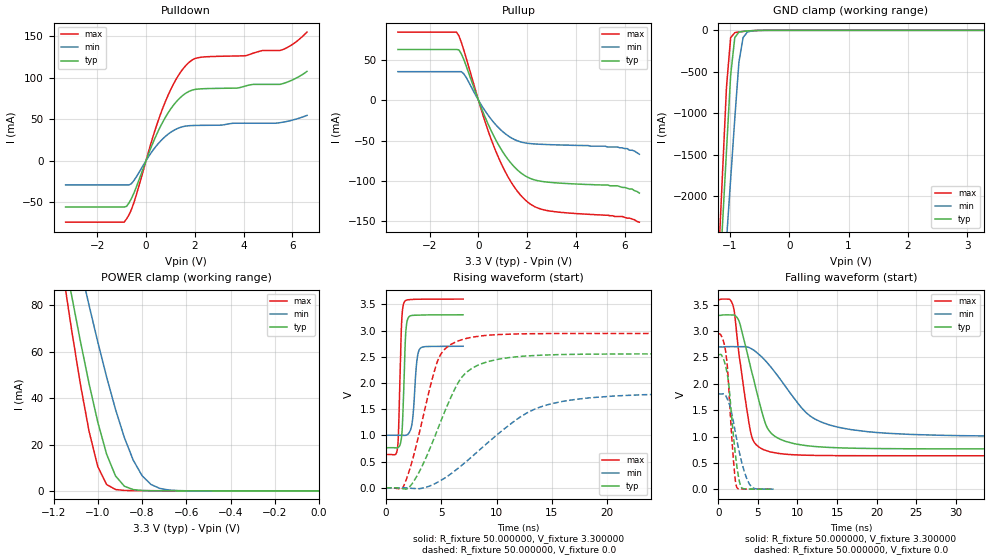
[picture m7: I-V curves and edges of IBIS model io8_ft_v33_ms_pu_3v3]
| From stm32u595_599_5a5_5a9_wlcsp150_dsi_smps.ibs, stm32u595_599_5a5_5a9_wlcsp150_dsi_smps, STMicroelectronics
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|   Model io8_ft_v33_ms_pu_3v3
[Model]  io8_ft_v33_ms_pu_3v3
Model_type I/O
Polarity   Non-Inverting
Enable   Active-Low
Vinl =   0.990000V
Vinh =   2.310000V
Vmeas =  1.650000V
Cref =   50.000000pF
Rref =   100.000000M
Vref =   0.0V
C_comp   3.252200pF   3.221000pF   3.293600pF
[Temperature Range]   25.000000   0.140000k   -40.000000
[Pullup Reference]   3.300000V   2.700000V   3.600000V
[Pulldown Reference]   0.0V   0.0V   0.0V
[POWER Clamp Reference]   3.300000V   2.700000V   3.600000V
[GND Clamp Reference]   0.0V   0.0V   0.0V
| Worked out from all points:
|   slope of the pulldown table from 0 to 0.495 V, typ, clamps not added: 14 ohm
|   slope of the pullup table from 0 to 0.495 V, typ, clamps not added: 13.7 ohm
|   GND clamp passes 1 mA (typ) near -0.51 V on its own axis
|   POWER clamp passes 1 mA (typ) near -0.85 V on its own axis
|   rising waveform, R_fixture 50.000000, V_fixture 3.300000: 20-80 % time 245ps typ, 337ps min, 229ps max; typ from 0.765 V to 3.3 V
|   rising waveform, R_fixture 50.000000, V_fixture 0.0: 20-80 % time 3.16ns typ, 6.46ns min, 2.09ns max; typ from 0.001 V to 2.55 V
|   falling waveform, R_fixture 50.000000, V_fixture 3.300000: 20-80 % time 2.58ns typ, 5.68ns min, 1.62ns max; typ from 3.3 V to 0.765 V
|   falling waveform, R_fixture 50.000000, V_fixture 0.0: 20-80 % time 1ns typ, 1.54ns min, 765ps max; typ from 2.55 V to 0.001 V
[Pulldown]
|Voltage   I(typ)   I(min)   I(max)
-3.3V     -56.06mA   -29.42mA   -74.35mA
-900mV    -56.06mA   -29.42mA   -74.35mA
-700mV    -51.09mA   -29.42mA   -65.48mA
-500mV    -39.32mA   -24.2mA    -50.88mA
300mV     22.62mA    13.13mA    30.42mA
800mV     52.54mA    29.36mA    71.75mA
1.3V      72.91mA    38.82mA    101.4mA
1.8V      84.02mA    42.13mA    119.4mA
2.3V      86.61mA    42.5mA     124.8mA
5.5V      91.96mA    45.75mA    132.9mA
6.1V      98.6mA     49.6mA     142.1mA
6.6V      107.6mA    54.5mA     155mA
[Pullup]
|Voltage   I(typ)   I(min)   I(max)
-3.3V     62.56mA    35.13mA    84.07mA
-900mV    62.56mA    35.13mA    84.07mA
-800mV    62.09mA    35.13mA    79.5mA
-600mV    50.25mA    32.46mA    61.91mA
200mV     -15.65mA   -9.933mA   -19.95mA
700mV     -48.51mA   -30.11mA   -62.22mA
1.3V      -76.68mA   -45.83mA   -99.4mA
1.6V      -86.41mA   -50.38mA   -112.8mA
2V        -95.1mA    -53.38mA   -125.6mA
2.8V      -101.3mA   -54.97mA   -136.5mA
5.7V      -106mA     -58mA      -144mA
6.6V      -115mA     -67mA      -151mA
[GND_clamp]
|Voltage   I(typ)   I(min)   I(max)
-3.3V     -9.848A    -9.957A    -9.458A
-1.2V     -3.312A    -4.013A    -2.863A
-1.13V    -2.381A    -3.274A    -1.769A
-1.06V    -1.452A    -2.535A    -684.7mA
-990mV    -542.9mA   -1.798A    -88.02mA
-920mV    -87.11mA   -1.064A    -28.44mA
-850mV    -22.1mA    -382.4mA   -19.61mA
-780mV    -11.97mA   -86.98mA   -13.71mA
-710mV    -7.619mA   -22.26mA   -8.745mA
-640mV    -4.493mA   -7.773mA   -4.817mA
-360mV    -31.22uA   -172.6uA   -8.607uA
3.28V     0A         15.66nA    -5.841nA
[POWER_clamp]
|Voltage   I(typ)   I(min)   I(max)
-3.28V    1.355A     1.167A     1.665A
-1.16V    105.8mA    131.6mA    95.87mA
-1.12V    85.09mA    114mA      70.46mA
-1.08V    65.2mA     96.88mA    46.75mA
-1.04V    46.48mA    80.2mA     25.96mA
-1V       29.64mA    64.18mA    10.49mA
-960mV    15.81mA    49.06mA    2.744mA
-920mV    6.482mA    35.16mA    613.3uA
-840mV    578.4uA    13.29mA    138.7uA
-760mV    94.46uA    2.808mA    98.68uA
-640mV    40.58uA    159.2uA    60uA
0V        0A         19.29nA    0A
[Ramp]
| variable   typ   min   max
dV/dt_r  1.53214/3.15170n   1.08393/6.44964n   1.76630/2.09040n
dV/dt_f  1.52095/2.57566n   1.01712/5.67238n   1.77908/1.61568n
R_load = 50.000000
[Rising Waveform]
R_fixture= 50.000000
V_fixture= 3.300000
V_fixture_min= 2.700000
V_fixture_max= 3.600000
|time   V(typ)   V(min)   V(max)
0s        765.1mV    1.003V     634.9mV
1.065ns   765.1mV    1.003V     780.8mV
1.415ns   964.6mV    1.002V     3.111V
1.654ns   2.115V     1V         3.538V
1.78ns    2.896V     1.002V     3.571V
1.948ns   3.201V     1.015V     3.584V
2.396ns   3.289V     1.272V     3.593V
2.775ns   3.292V     2.368V     3.596V
3.041ns   3.294V     2.641V     3.597V
6.979ns   3.3V       2.7V       3.6V
[Rising Waveform]
R_fixture= 50.000000
V_fixture= 0.0
V_fixture_min= 0.0
V_fixture_max= 0.0
|time   V(typ)   V(min)   V(max)
0s        861.5uV    874.5uV    909.2uV
1.441ns   -14.3mV    1.043mV    -20.16mV
2.432ns   96.28mV    -11.32mV   554.6mV
4.685ns   1.119V     108.2mV    2.424V
5.405ns   1.499V     197.7mV    2.661V
6.937ns   2.128V     443.5mV    2.83V
8.649ns   2.368V     757.6mV    2.898V
12.16ns   2.506V     1.354V     2.936V
16.04ns   2.543V     1.651V     2.943V
44.86ns   2.554V     1.808V     2.944V
[Falling Waveform]
R_fixture= 50.000000
V_fixture= 3.300000
V_fixture_min= 2.700000
V_fixture_max= 3.600000
|time   V(typ)   V(min)   V(max)
0s        3.3V       2.7V       3.6V
1.892ns   3.307V     2.706V     3.477V
2.703ns   3.159V     2.705V     2.479V
4.054ns   2.338V     2.678V     1.116V
5.676ns   1.383V     2.484V     753.4mV
6.396ns   1.117V     2.364V     716.9mV
7.748ns   953.7mV    2.104V     677.1mV
11.62ns   819.2mV    1.388V     643.5mV
15.23ns   785.8mV    1.174V     637.3mV
44.86ns   765.1mV    1.003V     634.9mV
[Falling Waveform]
R_fixture= 50.000000
V_fixture= 0.0
V_fixture_min= 0.0
V_fixture_max= 0.0
|time   V(typ)   V(min)   V(max)
0s        2.554V     1.808V     2.944V
560.6ps   2.507V     1.809V     2.856V
1.037ns   2.27V      1.749V     2.502V
1.345ns   1.972V     1.642V     1.895V
1.906ns   1.036V     1.292V     592.2mV
2.144ns   696.8mV    1.098V     191.1mV
2.298ns   505.5mV    975.8mV    56.66mV
2.831ns   65.58mV    595.8mV    4.018mV
3.938ns   2.984mV    96.69mV    1.774mV
6.979ns   861.5uV    874.5uV    909.2uV
